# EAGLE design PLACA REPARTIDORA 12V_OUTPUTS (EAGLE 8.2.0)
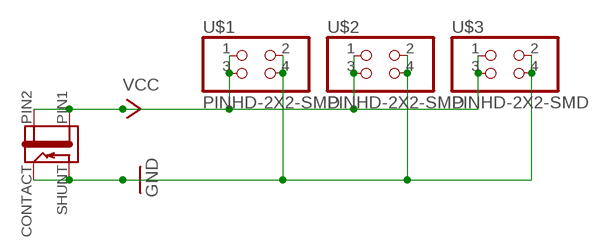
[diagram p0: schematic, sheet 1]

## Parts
J1  JACK-2.1MM  [PJ-002AH-SMT]
U$1  PINHD-2X2-SMD  [2X02SMD]
U$2  PINHD-2X2-SMD  [2X02SMD]
U$3  PINHD-2X2-SMD  [2X02SMD]

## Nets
GND: J1.CONTACT J1.SHUNT U$1.2 U$1.4 U$2.2 U$2.4 U$3.2 U$3.4
VCC: J1.PIN1 J1.PIN2 U$1.1 U$1.3 U$2.1 U$2.3 U$3.1 U$3.3

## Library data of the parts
J1 = fab:JACK-2.1MM: SMD DC power jack PJ-002AH-SMT As found in the fablab inventory. Made by Zaerc.
U$1-U$3 = fab:PINHD-2X2-SMD

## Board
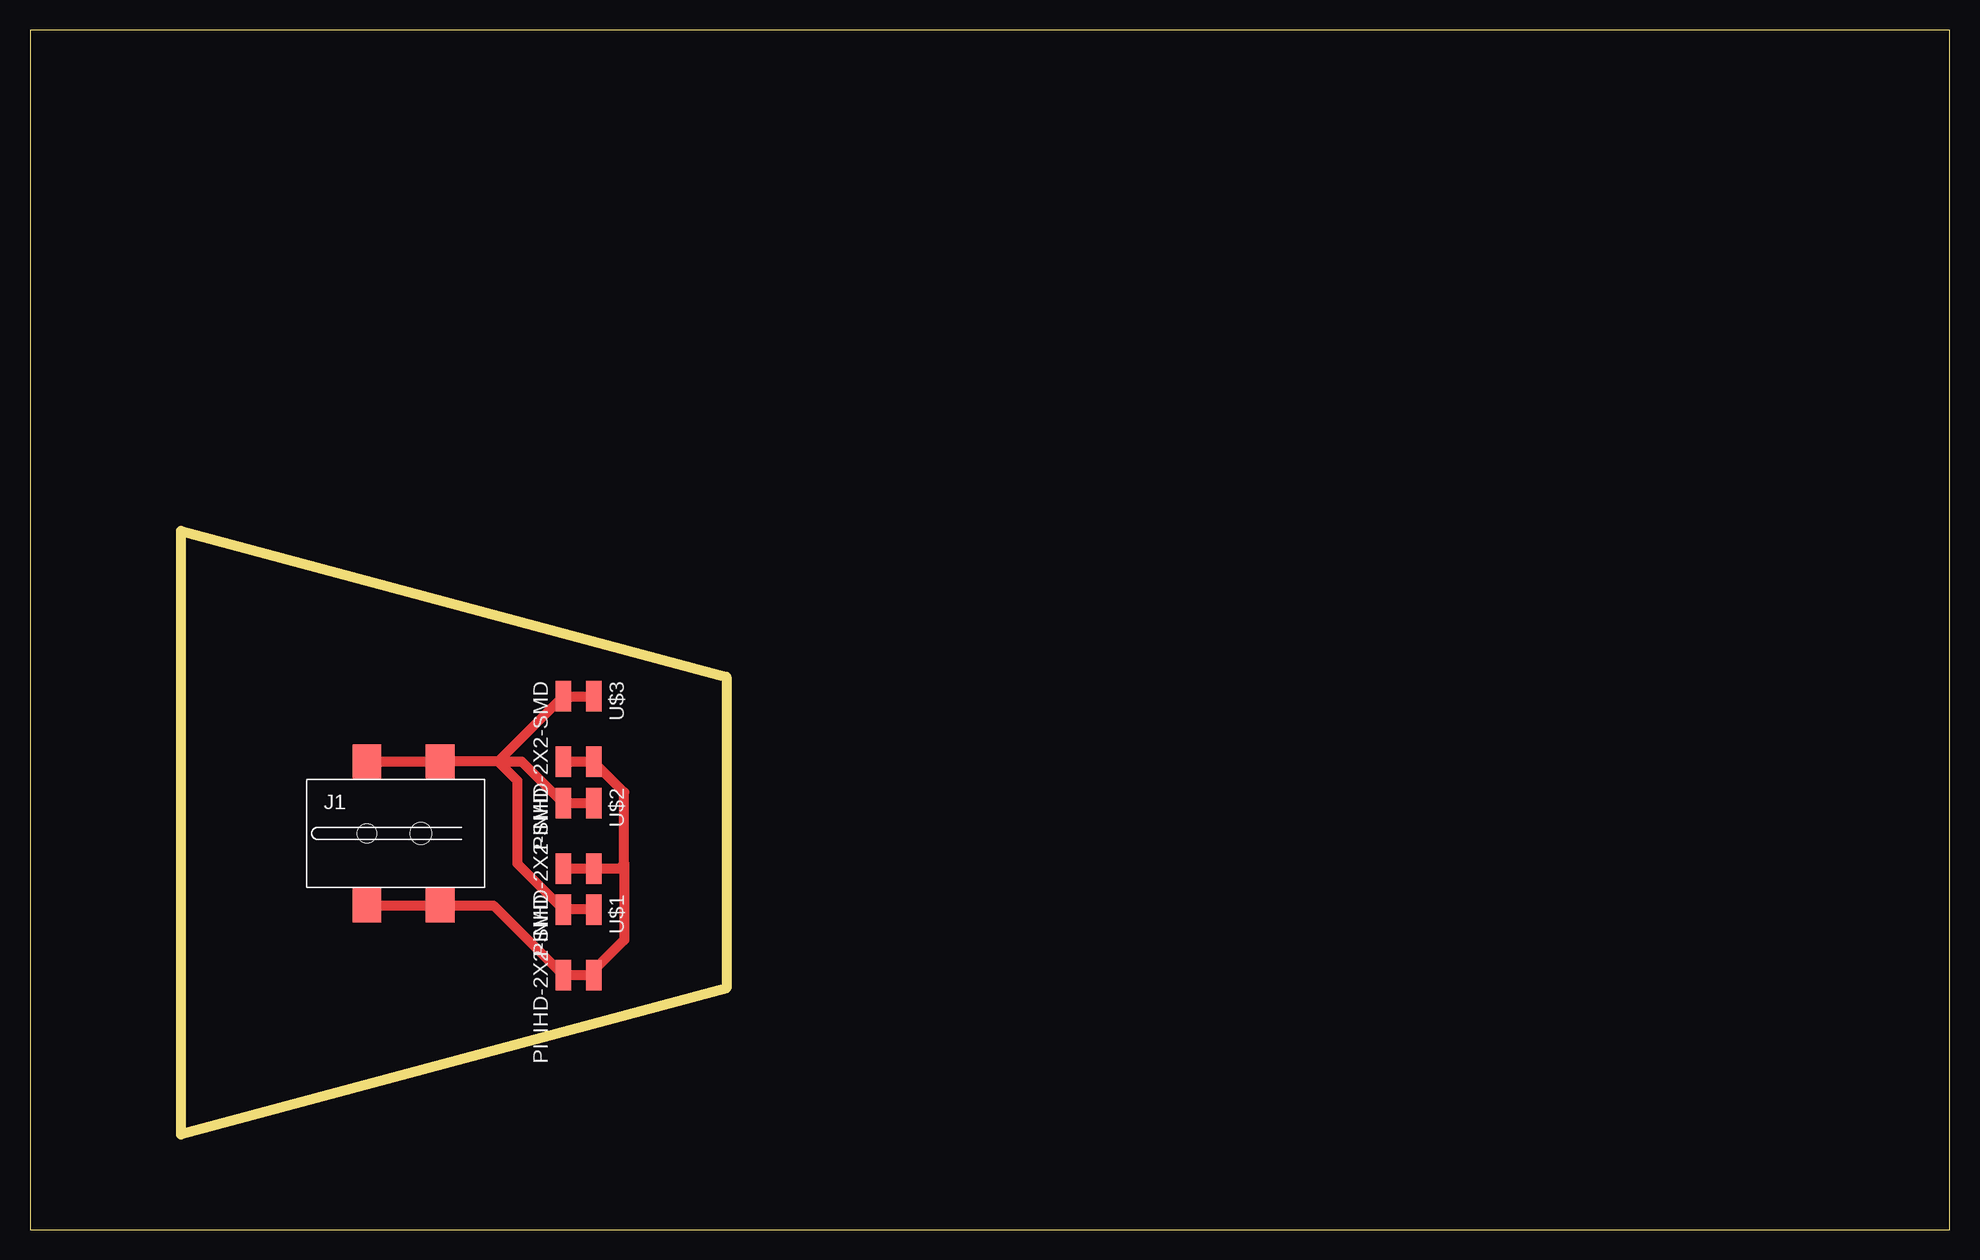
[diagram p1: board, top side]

Size 160 x 100 mm. Coordinates in mm from the lower left corner, seen from the top.
Outline: 0,0 160,0 160,100 0,100 0,0
Outline: 58.05,20.12 12.59,7.94 12.59,58.25 58.05,46.06 58.05,20.12
Copper layers (1*16): Top 0.035mm / dielectric 1.5mm / Bottom 0.035mm
Design rules "default": minimum track width 6mil, minimum drill 0.35mm, track to track 6mil, track to pad 6mil, pad to pad 6mil, via to via 6mil, smd to smd 6mil, copper to edge 40mil, drill to drill 6mil, minimum pad ring 10mil, minimum via ring 8mil, stop-mask expansion 4mil, vias tented up to drill 0mil, thermal gap 10mil

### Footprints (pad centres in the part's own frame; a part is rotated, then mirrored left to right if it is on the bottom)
PJ-002AH-SMT = smd 2.4 x 2.8: CONTACT -2.4,-6; PIN1 3.7,6; PIN2 -2.4,6; SHUNT 3.7,-6 | hole 1.6: -2.4,0 | hole 1.8: 2.1,0
2X02SMD = smd 2.54 x 1.27: 1 -2.54,1.27; 2 2.92,1.27; 3 -2.54,-1.27; 4 2.92,-1.27

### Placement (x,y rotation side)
J1  30.48,33.02 0 top
U$1  45.72,24.13 270 top
U$2  45.72,33.02 270 top
U$3  45.72,41.91 270 top

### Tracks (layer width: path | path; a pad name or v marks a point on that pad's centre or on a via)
GND
  Top 0.813: J1.CONTACT J1.SHUNT 38.64,27.02 U$1.4 U$1.2 46.99,21.59 49.53,24.13 49.53,30.48 | U$3.4 U$3.2 49.53,36.45 49.53,30.48 | U$2.4 U$2.2 49.15,30.1 49.53,30.48
VCC
  Top 0.813: J1.PIN2 J1.PIN1 39.02,39.02 | 39.02,39.02 U$3.3 U$3.1 | 39.02,39.02 40.99,39.02 U$2.3 U$2.1 | U$1.1 U$1.3 40.64,30.48 40.64,37.4 39.02,39.02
